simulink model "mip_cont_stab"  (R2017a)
settings: Solver=VariableStepAuto  StartTime=0.0  StopTime=50.0  RelTol=1e-3
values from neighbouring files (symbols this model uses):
  g = 9.81    [analisi_linearizzato.m]
  Ir = 10    [analisi_linearizzato.m]
  Iw = 0.06    [analisi_linearizzato.m]
  L = 0.4    [analisi_linearizzato.m]
  mr = 3    [analisi_linearizzato.m]
  mw = 20    [analisi_linearizzato.m]
  R = 0.2    [analisi_linearizzato.m]
  R1 = zpk(P_G1{1}(2),P_G1{1}(2)-4,(2+P_G1{1}(1))^2/K_G1)    [analisi_linearizzato.m]
undefined symbols (not defined in the file or in its folder): magnitude

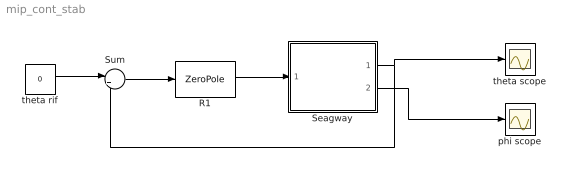
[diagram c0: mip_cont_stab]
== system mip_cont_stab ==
  R1 : ZeroPole  Zeros=R1.z{1}  Poles=R1.p{1}  Gain=R1.k
  Seagway : Subsystem
  Sum : Sum  Inputs=|+-
  phi scope : Scope
  theta rif : Constant  Value=0
  theta scope : Scope
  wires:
  Sum/1 -> R1/1
  R1/1 -> Seagway/1(Tau)
  Seagway/1(Theta) -> Sum/2, theta scope/1
  Seagway/2(Phi) -> phi scope/1
  theta rif/1 -> Sum/1

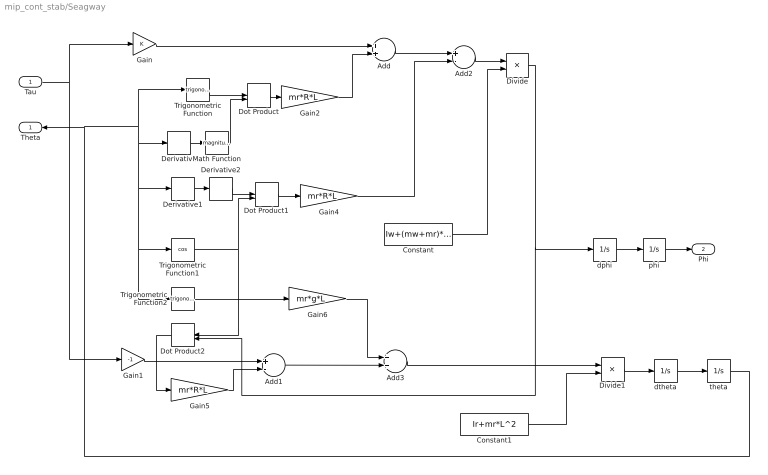
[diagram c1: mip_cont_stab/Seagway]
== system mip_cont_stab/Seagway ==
  Tau : Inport
  Add : Sum
  Add1 : Sum  Inputs=+-
  Add2 : Sum  Inputs=+-
  Add3 : Sum
  Constant : Constant  Value=Iw+(mw+mr)*R^2
  Constant1 : Constant  Value=Ir+mr*L^2
  Derivative : Derivative
  Derivative1 : Derivative
  Derivative2 : Derivative
  Divide : Product  Inputs=*/
  Divide1 : Product  Inputs=*/
  Dot Product : DotProduct
  Dot Product1 : DotProduct
  Dot Product2 : DotProduct
  Gain : Gain
  Gain1 : Gain  Gain=-1
  Gain2 : Gain  Gain=mr*R*L
  Gain4 : Gain  Gain=mr*R*L
  Gain5 : Gain  Gain=mr*R*L
  Gain6 : Gain  Gain=mr*g*L
  Math Function : Math  Operator=magnitude^2
  Trigonometric Function : Trigonometry
  Trigonometric Function1 : Trigonometry  Operator=cos
  Trigonometric Function2 : Trigonometry
  dphi : Integrator
  dtheta : Integrator
  phi : Integrator
  theta : Integrator
  Theta : Outport
  Phi : Outport  Port=2
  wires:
  Add1/1 -> Add3/2
  phi/1 -> Phi/1
  dphi/1 -> phi/1
  Divide1/1 -> dtheta/1
  dtheta/1 -> theta/1
  Derivative2/1 -> Dot Product1/1
  Add/1 -> Add2/1
  Divide/1 -> Dot Product2/2, dphi/1
  Derivative/1 -> Math Function/1
  Dot Product1/1 -> Gain4/1
  Trigonometric Function1/1 -> Dot Product1/2, Dot Product2/1
  Derivative1/1 -> Derivative2/1
  theta/1 -> Trigonometric Function1/1, Trigonometric Function2/1, Derivative1/1, Derivative/1, Trigonometric Function/1, Theta/1
  Math Function/1 -> Dot Product/2
  Add2/1 -> Divide/1
  Gain5/1 -> Add1/2
  Constant/1 -> Divide/2
  Gain1/1 -> Add1/1
  Add3/1 -> Divide1/1
  Dot Product2/1 -> Gain5/1
  Trigonometric Function/1 -> Dot Product/1
  Tau/1 -> Gain/1, Gain1/1
  Gain4/1 -> Add2/2
  Trigonometric Function2/1 -> Gain6/1
  Dot Product/1 -> Gain2/1
  Gain6/1 -> Add3/1
  Gain2/1 -> Add/2
  Gain/1 -> Add/1
  Constant1/1 -> Divide1/2
